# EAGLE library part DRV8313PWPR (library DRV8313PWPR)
2.5A Three Phase Brushless DC Motor Driver (PWM Ctrl) Source: Datasheet
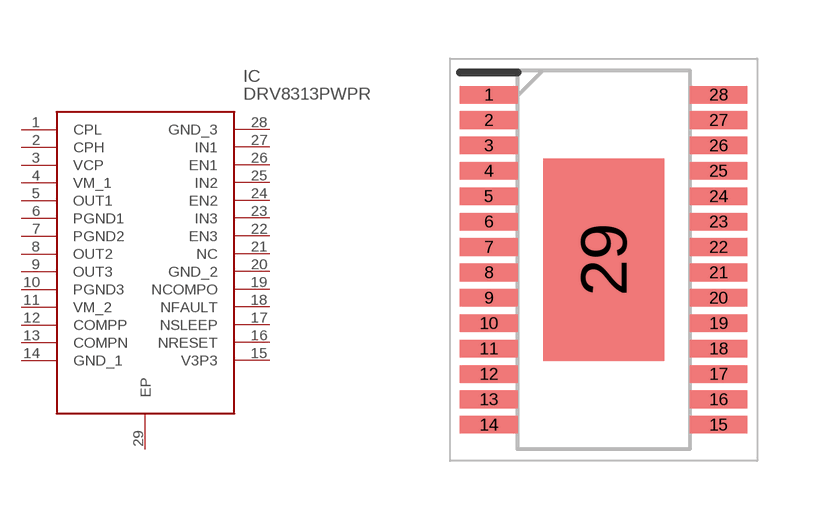
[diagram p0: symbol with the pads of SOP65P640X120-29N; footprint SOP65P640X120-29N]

Designator prefix IC

## DRV8313PWPR (Arrow_Part_Number: DRV8313PWPR; Arrow_Price-Stock: https://www.arrow.com/en/products/drv8313pwpr/texas-instruments?region=nac; Description: 2.5A Three Phase Brushless DC Motor Driver (PWM Ctrl); Height: 1.2mm; Manufacturer_Name: Texas Instruments; Manufacturer_Part_Number: DRV8313PWPR; Mouser_Part_Number: 595-DRV8313PWPR; Mouser_Price-Stock: https://www.mouser.co.uk/ProductDetail/Texas-Instruments/DRV8313PWPR?qs=aQEsdMNF%2FMwPk4783CnTRg%3D%3D)  [SOP65P640X120-29N]
1  CPL
2  CPH
3  VCP
4  VM_1
5  OUT1
6  PGND1
7  PGND2
8  OUT2
9  OUT3
10  PGND3
11  VM_2
12  COMPP
13  COMPN
14  GND_1
15  V3P3
16  NRESET
17  NSLEEP
18  NFAULT
19  NCOMPO
20  GND_2
21  NC  nc
22  EN3
23  IN3
24  EN2
25  IN2
26  EN1
27  IN1
28  GND_3
29  EP

## Footprint SOP65P640X120-29N (pad centres in mm)
PWP
smd 1.475 x 0.45: 1 -2.938,4.225; 2 -2.938,3.575; 3 -2.938,2.925; 4 -2.938,2.275; 5 -2.938,1.625; 6 -2.938,0.975; 7 -2.938,0.325; 8 -2.938,-0.325; 9 -2.938,-0.975; 10 -2.938,-1.625; 11 -2.938,-2.275; 12 -2.938,-2.925; 13 -2.938,-3.575; 14 -2.938,-4.225; 15 2.938,-4.225; 16 2.938,-3.575; 17 2.938,-2.925; 18 2.938,-2.275; 19 2.938,-1.625; 20 2.938,-0.975; 21 2.938,-0.325; 22 2.938,0.325; 23 2.938,0.975; 24 2.938,1.625; 25 2.938,2.275; 26 2.938,2.925; 27 2.938,3.575; 28 2.938,4.225
smd 3.1 x 5.18: 29 0,0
